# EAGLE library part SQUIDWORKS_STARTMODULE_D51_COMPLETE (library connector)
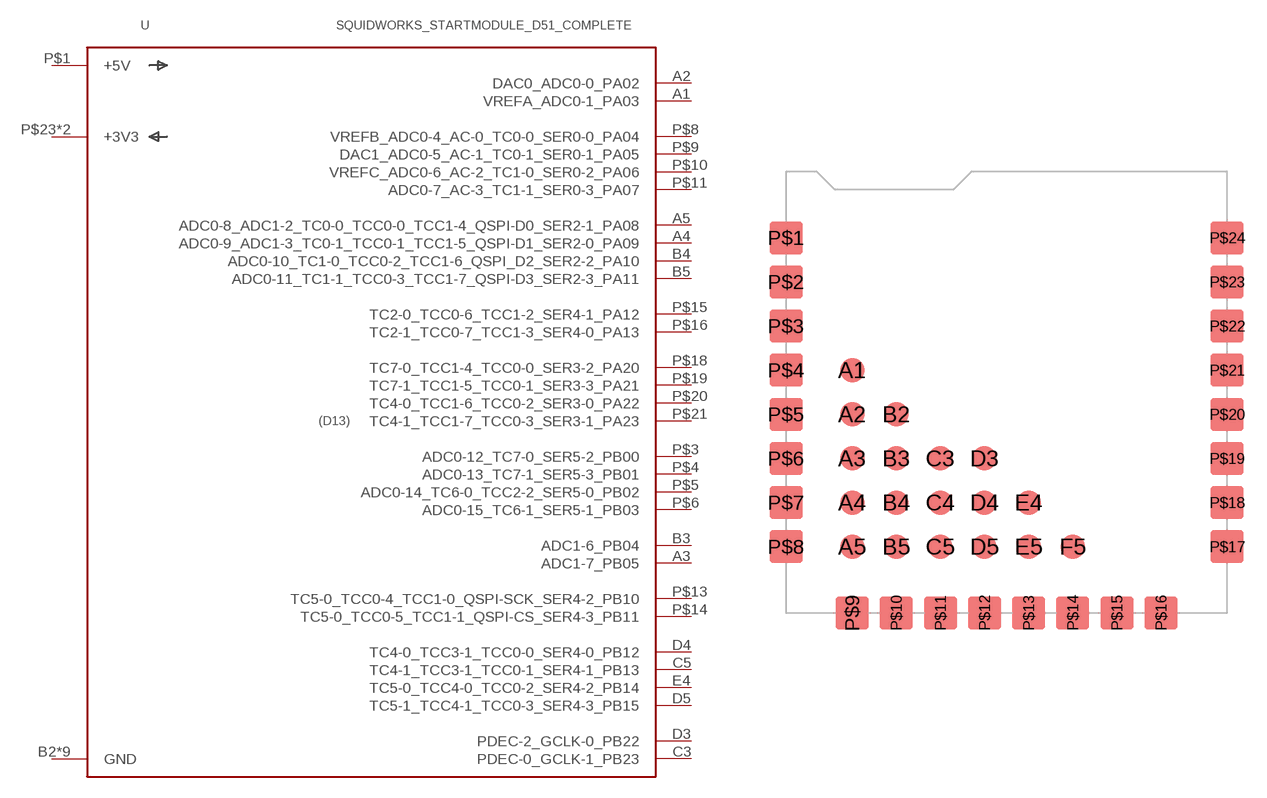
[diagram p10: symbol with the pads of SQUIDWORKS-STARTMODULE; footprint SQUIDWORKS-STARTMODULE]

Designator prefix U

## SQUIDWORKS_STARTMODULE_D51_COMPLETE  [SQUIDWORKS-STARTMODULE]
A1  VREFA_ADC0-1_PA03
A2  DAC0_ADC0-0_PA02
A3  ADC1-7_PB05
A4  ADC0-9_ADC1-3_TC0-1_TCC0-1_TCC1-5_QSPI-D1_SER2-0_PA09
A5  ADC0-8_ADC1-2_TC0-0_TCC0-0_TCC1-4_QSPI-D0_SER2-1_PA08
B2  GND
B3  ADC1-6_PB04
B4  ADC0-10_TC1-0_TCC0-2_TCC1-6_QSPI_D2_SER2-2_PA10
B5  ADC0-11_TC1-1_TCC0-3_TCC1-7_QSPI-D3_SER2-3_PA11
C3  PDEC-0_GCLK-1_PB23
C4  GND
C5  TC4-1_TCC3-1_TCC0-1_SER4-1_PB13
D3  PDEC-2_GCLK-0_PB22
D4  TC4-0_TCC3-1_TCC0-0_SER4-0_PB12
D5  TC5-1_TCC4-1_TCC0-3_SER4-3_PB15
E4  TC5-0_TCC4-0_TCC0-2_SER4-2_PB14
E5  GND
F5  GND
P$1  +5V
P$2  GND
P$3  ADC0-12_TC7-0_SER5-2_PB00
P$4  ADC0-13_TC7-1_SER5-3_PB01
P$5  ADC0-14_TC6-0_TCC2-2_SER5-0_PB02
P$6  ADC0-15_TC6-1_SER5-1_PB03
P$7  GND
P$8  VREFB_ADC0-4_AC-0_TC0-0_SER0-0_PA04
P$9  DAC1_ADC0-5_AC-1_TC0-1_SER0-1_PA05
P$10  VREFC_ADC0-6_AC-2_TC1-0_SER0-2_PA06
P$11  ADC0-7_AC-3_TC1-1_SER0-3_PA07
P$12  GND
P$13  TC5-0_TCC0-4_TCC1-0_QSPI-SCK_SER4-2_PB10
P$14  TC5-0_TCC0-5_TCC1-1_QSPI-CS_SER4-3_PB11
P$15  TC2-0_TCC0-6_TCC1-2_SER4-1_PA12
P$16  TC2-1_TCC0-7_TCC1-3_SER4-0_PA13
P$17  GND
P$18  TC7-0_TCC1-4_TCC0-0_SER3-2_PA20
P$19  TC7-1_TCC1-5_TCC0-1_SER3-3_PA21
P$20  TC4-0_TCC1-6_TCC0-2_SER3-0_PA22
P$21  TC4-1_TCC1-7_TCC0-3_SER3-1_PA23
P$22  GND
P$23  +3V3
P$24  +3V3

## Footprint SQUIDWORKS-STARTMODULE (pad centres in mm)
smd 1.397 x 1.397: A1 -8.89,1.27; A2 -8.89,-1.27; A3 -8.89,-3.81; A4 -8.89,-6.35; A5 -8.89,-8.89; B2 -6.35,-1.27; B3 -6.35,-3.81; B4 -6.35,-6.35; B5 -6.35,-8.89; C3 -3.81,-3.81; C4 -3.81,-6.35; C5 -3.81,-8.89; D3 -1.27,-3.81; D4 -1.27,-6.35; D5 -1.27,-8.89; E4 1.27,-6.35; E5 1.27,-8.89; F5 3.81,-8.89
smd 1.905 x 1.905: P$1 -12.7,8.89; P$2 -12.7,6.35; P$3 -12.7,3.81; P$4 -12.7,1.27; P$5 -12.7,-1.27; P$6 -12.7,-3.81; P$7 -12.7,-6.35; P$8 -12.7,-8.89; P$9 -8.89,-12.7; P$10 -6.35,-12.7; P$11 -3.81,-12.7; P$12 -1.27,-12.7; P$13 1.27,-12.7; P$14 3.81,-12.7; P$15 6.35,-12.7; P$16 8.89,-12.7; P$17 12.7,-8.89; P$18 12.7,-6.35; P$19 12.7,-3.81; P$20 12.7,-1.27; P$21 12.7,1.27; P$22 12.7,3.81; P$23 12.7,6.35; P$24 12.7,8.89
